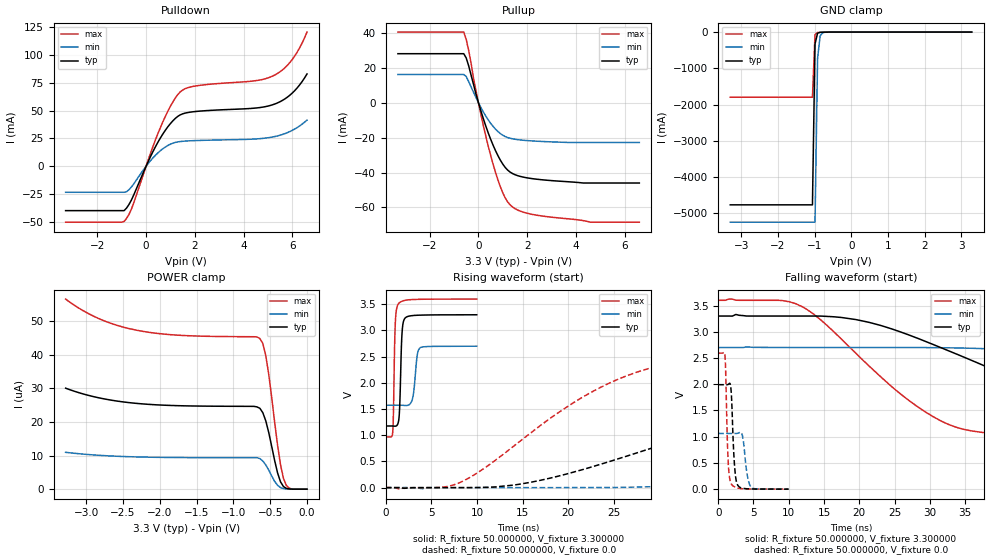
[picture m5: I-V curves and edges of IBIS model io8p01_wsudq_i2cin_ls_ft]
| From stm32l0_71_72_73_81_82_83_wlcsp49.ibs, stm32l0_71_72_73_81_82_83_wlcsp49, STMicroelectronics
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|   Model io8p01_wsudq_i2cin_ls_ft
[Model]  io8p01_wsudq_i2cin_ls_ft
Model_type I/O
Polarity   Non-Inverting
Enable   Active-Low
Vinl =   0.990000V
Vinh =   2.310000V
Vmeas =  1.650000V
Cref =   50.000000pF
Rref =   100.000000M
Vref =   0.0V
C_comp   3.020400pF   2.988200pF   3.054500pF
[Temperature Range]   25.000000   0.125000k   -40.000000
[Pullup Reference]   3.300000V   2.700000V   3.600000V
[Pulldown Reference]   0.0V   0.0V   0.0V
[POWER Clamp Reference]   3.300000V   2.700000V   3.600000V
[GND Clamp Reference]   0.0V   0.0V   0.0V
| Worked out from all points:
|   slope of the pulldown table from 0 to 0.495 V, typ, clamps not added: 22.6 ohm
|   slope of the pullup table from 0 to 0.495 V, typ, clamps not added: 23.9 ohm
|   GND clamp passes 1 mA (typ) near -0.64 V on its own axis
|   rising waveform, R_fixture 50.000000, V_fixture 3.300000: 20-80 % time 222ps typ, 369ps min, 182ps max; typ from 1.18 V to 3.3 V
|   rising waveform, R_fixture 50.000000, V_fixture 0.0: 20-80 % time 27.1ns typ, 59.5ns min, 13.6ns max; typ from 0 V to 1.99 V
|   falling waveform, R_fixture 50.000000, V_fixture 3.300000: 20-80 % time 24.2ns typ, 53.4ns min, 13.3ns max; typ from 3.3 V to 1.18 V
|   falling waveform, R_fixture 50.000000, V_fixture 0.0: 20-80 % time 406ps typ, 572ps min, 327ps max; typ from 1.99 V to 0 V
[Pulldown]
|Voltage   I(typ)   I(min)   I(max)
-3.3V     -39.83mA   -23.37mA   -50.21mA
-900mV    -39.83mA   -23.37mA   -49.53mA
-600mV    -30.28mA   -18.59mA   -38.45mA
500mV     22.11mA    12.28mA    30.1mA
1V        38.33mA    19.81mA    53.88mA
1.4V      46.1mA     22.18mA    66.72mA
2V        49.07mA    23.02mA    71.93mA
4.4V      52.05mA    24.38mA    76.53mA
5.2V      55.25mA    26.31mA    81.02mA
5.6V      59.18mA    28.57mA    86.57mA
6V        65.79mA    32.24mA    95.97mA
6.6V      82.83mA    41.41mA    120.4mA
[Pullup]
|Voltage   I(typ)   I(min)   I(max)
-3.3V     27.97mA    16.08mA    40.34mA
-600mV    27.97mA    16.08mA    40.34mA
-400mV    21.07mA    12.09mA    29.9mA
-200mV    10.4mA     5.946mA    13.84mA
200mV     -9.115mA   -5.294mA   -12.98mA
600mV     -24.29mA   -13.56mA   -35.12mA
1V        -35.2mA    -18.69mA   -51.63mA
1.2V      -38.62mA   -20mA      -56.79mA
1.4V      -40.6mA    -20.72mA   -59.71mA
2.2V      -43.48mA   -21.92mA   -63.91mA
4.6V      -46mA      -22.8mA    -68.41mA
6.6V      -46mA      -22.8mA    -68.41mA
[GND_clamp]
|Voltage   I(typ)   I(min)   I(max)
-3.3V     -4.766A    -5.244A    -1.797A
-1.06V    -4.766A    -5.244A    -1.797A
-990mV    -326.6mA   -5.244A    -67.9mA
-920mV    -28.92mA   -722.1mA   -10.96mA
-850mV    -6.612mA   -104.2mA   -6.532mA
-780mV    -3.464mA   -17.27mA   -4.209mA
-500mV    -57.88uA   -167.8uA   -34.02uA
3.28V     0A         0A         0A
[POWER_clamp]
|Voltage   I(typ)   I(min)   I(max)
-3.28V    30.07uA    10.97uA    56.59uA
-2.84V    27.25uA    10.1uA     50.89uA
-2.32V    25.55uA    9.602uA    47.34uA
-640mV    24.06uA    9.099uA    44.84uA
-600mV    22.76uA    8.364uA    43.37uA
-560mV    20.32uA    7.211uA    39.74uA
-520mV    16.86uA    5.675uA    34.14uA
-400mV    4.841uA    1.145uA    13.1uA
-360mV    2.184uA    477.2nA    7.288uA
-320mV    772.4nA    180.3nA    3.213uA
-240mV    60.03nA    0A         295.3nA
0V        0A         0A         0A
[Ramp]
| variable   typ   min   max
dV/dt_r  1.19496/27.02727n   0.63570/59.48302n   1.55568/13.55602n
dV/dt_f  1.27416/24.18424n   0.67062/53.31860n   1.57856/13.28631n
R_load = 50.000000
[Rising Waveform]
R_fixture= 50.000000
V_fixture= 3.300000
V_fixture_min= 2.700000
V_fixture_max= 3.600000
|time   V(typ)   V(min)   V(max)
0s        1.176V     1.573V     969.1mV
740.7ps   1.176V     1.573V     1.038V
1.021ns   1.173V     1.573V     3.073V
1.361ns   1.243V     1.574V     3.506V
1.522ns   1.566V     1.574V     3.534V
1.782ns   2.965V     1.572V     3.559V
2.102ns   3.236V     1.568V     3.576V
2.903ns   3.284V     1.685V     3.59V
3.764ns   3.293V     2.67V      3.595V
9.97ns    3.3V       2.7V       3.6V
[Rising Waveform]
R_fixture= 50.000000
V_fixture= 0.0
V_fixture_min= 0.0
V_fixture_max= 0.0
|time   V(typ)   V(min)   V(max)
0s        -400nV     -2.238uV   -176.4nV
8.008ns   -464.7uV   -172.4uV   87.17mV
15.02ns   75.12mV    -160.7uV   924.7mV
24.52ns   496.4mV    2.89mV     1.994V
31.03ns   854.1mV    24.37mV    2.366V
38.54ns   1.216V     69.57mV    2.517V
57.56ns   1.756V     279.6mV    2.585V
81.58ns   1.946V     586.7mV    2.592V
137.1ns   1.991V     964.2mV    2.593V
249.2ns   1.992V     1.062V     2.593V
[Falling Waveform]
R_fixture= 50.000000
V_fixture= 3.300000
V_fixture_min= 2.700000
V_fixture_max= 3.600000
|time   V(typ)   V(min)   V(max)
0s        3.3V       2.7V       3.6V
12.01ns   3.3V       2.7V       3.472V
19.52ns   3.233V     2.7V       2.589V
29.03ns   2.835V     2.699V     1.502V
39.04ns   2.276V     2.671V     1.061V
56.06ns   1.484V     2.524V     988mV
72.07ns   1.283V     2.31V      975mV
104.1ns   1.201V     1.874V     969.9mV
133.1ns   1.183V     1.701V     969.2mV
249.2ns   1.176V     1.573V     969.1mV
[Falling Waveform]
R_fixture= 50.000000
V_fixture= 0.0
V_fixture_min= 0.0
V_fixture_max= 0.0
|time   V(typ)   V(min)   V(max)
0s        1.992V     1.062V     2.593V
961ps     1.992V     1.062V     2.541V
1.401ns   1.996V     1.062V     567.8mV
1.842ns   1.856V     1.062V     105.2mV
2.302ns   477.3mV    1.061V     45.86mV
2.763ns   77.64mV    1.065V     21.64mV
3.423ns   18.91mV    1.027V     7.607mV
4.084ns   7.458mV    296.4mV    4.386mV
4.705ns   3.89mV     33.7mV     2.984mV
9.97ns    -400nV     -2.238uV   -176.4nV
